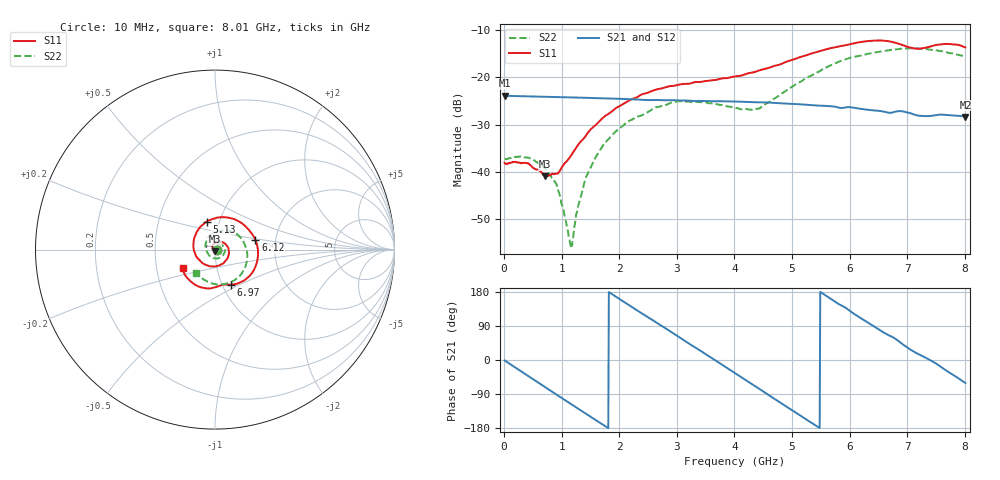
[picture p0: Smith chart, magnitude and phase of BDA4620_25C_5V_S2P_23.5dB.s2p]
!Agilent Technologies,E5071B,MY42404982,A.09.10
!Date: Wed May 06 09:03:28 2026
!Data & Calibration Information:
!Freq	S11:SOLT2(ON)	S21:SOLT2(ON)	S12:SOLT2(ON)	S22:SOLT2(ON)
# Hz S RI R 50
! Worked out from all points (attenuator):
!   801 points, 10 MHz to 8.01 GHz, reference 50 ohm
!   highest |S21| = -23.90 dB at 10 MHz (marker M1); lowest = -28.4 dB at 8.01 GHz (marker M2)
!   lowest |S11| = -40.9 dB at 710 MHz (marker M3), VSWR 1.02, Z = 50 - j0.896 ohm
!   |S11| at or under -10 dB: start of sweep to end of sweep
!   |S22| runs from -55.7 to -13.9 dB; largest |S21 - S12| = 0.00028
!   S11 on the Smith chart (normalised r, x): 10 MHz: 1.03, -0.00; 5.13 GHz: 0.87, +0.28; 6.12 GHz: 1.57, +0.18; 6.97 GHz: 1.10, -0.45; 8.01 GHz: 0.68, -0.14
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1e7  0.0125 -0.000778  0.0638 -0.00134  0.0639 -0.00138  0.0136 -0.00044
4e8  0.00952 -0.00798  0.0479 -0.0408  0.048 -0.0409  0.0135 -0.00442
7.1e8  -0.000129 -0.00897  0.02 -0.0591  0.02 -0.0592  0.0085 -0.00684
9.3e8  -0.00813 -0.00504  -0.00339 -0.0618  -0.00349 -0.0619  0.00351 -0.00586
1.16e9  -0.0139 0.00491  -0.0268 -0.0551  -0.027 -0.0552  -0.00143 -0.000812
1.19e9  -0.0144 0.0065  -0.0296 -0.0536  -0.0297 -0.0536  -0.00188 4.07e-05
1.27e9  -0.015 0.0111  -0.0366 -0.0488  -0.0367 -0.0489  -0.00305 0.00231
1.35e9  -0.0148 0.0157  -0.0428 -0.0432  -0.0429 -0.0432  -0.00346 0.00489
1.53e9  -0.0107 0.027  -0.0535 -0.028  -0.0536 -0.028  -0.0032 0.0116
1.77e9  0.00198 0.0394  -0.0596 -0.00418  -0.0597 -0.00419  0.000992 0.0207
2.15e9  0.0348 0.0437  -0.0491 0.0323  -0.0492 0.0324  0.0174 0.0293
2.68e9  0.075 0.00573  -0.00544 0.0572  -0.00539 0.0572  0.0446 0.0192
3.07e9  0.0709 -0.0457  0.0307 0.0481  0.0308 0.0481  0.0556 -0.00679
4.01e9  -0.0672 -0.0768  0.0456 -0.0315  0.0456 -0.0316  -0.0109 -0.0466
4.43e9  -0.118 -0.00167  0.0132 -0.0527  0.0132 -0.0528  -0.0453 -0.0114
5.13e9  -0.0471 0.1557  -0.0426 -0.0295  -0.0427 -0.0294  -0.0141 0.0875
5.35e9  0.0155 0.1787  -0.0494 -0.0115  -0.0495 -0.0115  0.0233 0.1026
6.12e9  0.2255 0.0528  -0.0218 0.0418  -0.0218 0.0419  0.1621 0.0375
6.68e9  0.1805 -0.1586  0.0177 0.0383  0.0178 0.0385  0.1706 -0.0905
6.97e9  0.0877 -0.195  0.0346 0.0254  0.0347 0.0254  0.1308 -0.1535
7.6e9  -0.0728 -0.2117  0.038 -0.0136  0.038 -0.0136  -0.0231 -0.1873
8.01e9  -0.181 -0.0998  0.0186 -0.0333  0.0187 -0.0334  -0.1036 -0.1279
